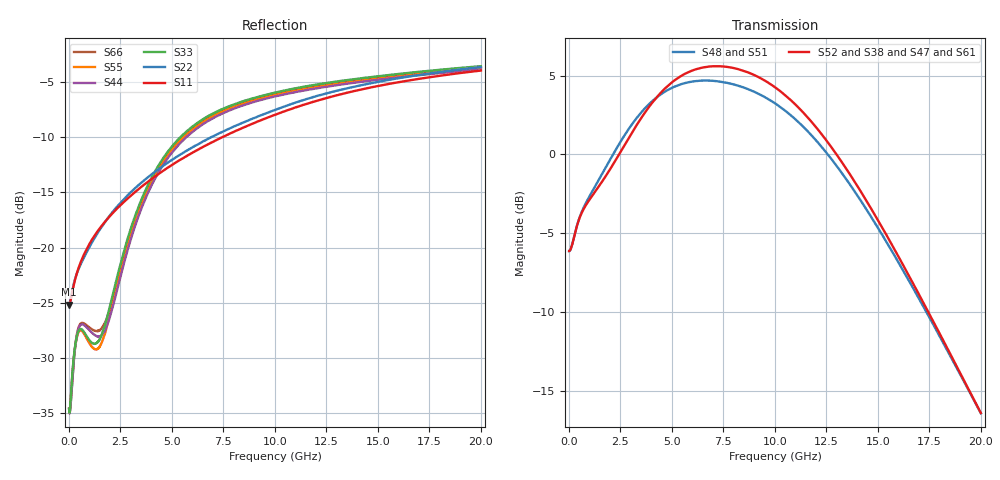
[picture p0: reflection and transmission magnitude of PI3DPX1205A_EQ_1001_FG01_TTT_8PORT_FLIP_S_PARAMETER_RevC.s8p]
! NPort=8 DATA=2000 NOISE=0 GROUPDELAY=0 COMPLEX_DATAFORMAT=POLAR
! NumOfBlock=1 NumOfParam=0
! .MODEL Smodel S TSTONEFILE=PI3DPX1205A_EQ_1001_FG01_TTT_8PORT_FLIP_S_PARAMETER_RevC.s8p TYPE=S
!  -- The above .MODEL line can be used for the S element in the netlist.
! The s parameter is extracted from the linear redriver, it is not bi-directional;
! only s(5,1)s(6,2)s(3,7)s(4,8) should be the insertion loss
!  Port definition:
!  Port1 = AIP
!  Port2 = AIN
!  Port3 = BOP
!  Port4 = BON
!  Port5 = AOP
!  Port6 = AON
!  Port7 = BIP
!  Port8 = BIN
# Hz S MA R  50
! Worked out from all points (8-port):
!   2000 points, 10 MHz to 20 GHz, reference 50 ohm
!   strongest paths, dB at 10 MHz, 5.01 GHz, 10.01 GHz, 15.01 GHz, 20 GHz:
!     S52: -6.1, 4.6, 4.3, -4.2, -16.4
!     S38: -6.1, 4.6, 4.2, -4.2, -16.4
!     S47: -6.1, 4.6, 4.3, -4.2, -16.4
!     S61: -6.1, 4.6, 4.3, -4.2, -16.4
!     S48: -6.1, 4.2, 3.2, -4.7, -16.4
!     S51: -6.1, 4.2, 3.2, -4.7, -16.4
!   lowest |S11| = -25.2 dB at 10 MHz (marker M1), VSWR 1.12, Z = 44.8 - j0.115 ohm
!   |S11| at or under -10 dB: start of sweep to 7.459 GHz
